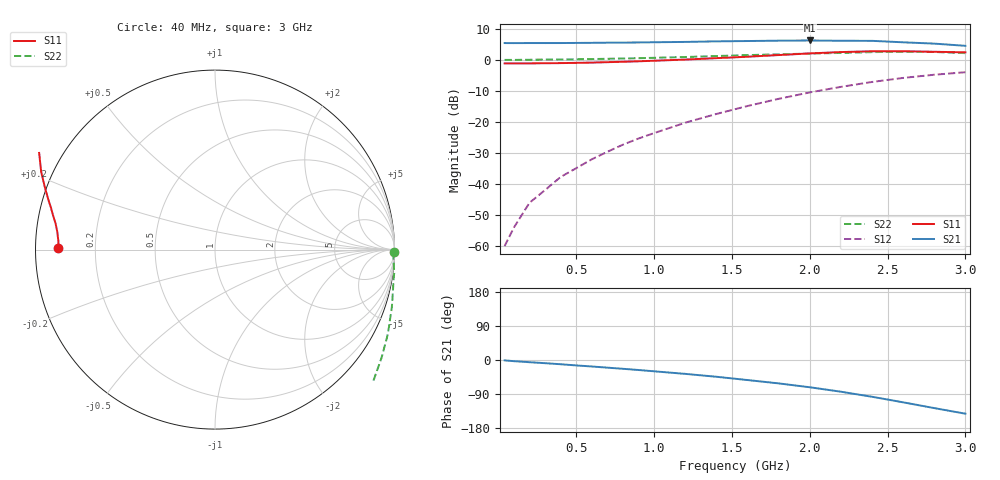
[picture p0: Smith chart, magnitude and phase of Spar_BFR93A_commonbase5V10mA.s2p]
! Filename:  BFR93ACB.S2P  Version:  2.0
! NXP part #: BFR93A  Date: Jul 1990
! Bias condition: Vce=5V, Ic=10mA
! COMMON BASE
#  MHz  S  MA  R  50
! Freq  S11  S21  S12  S22
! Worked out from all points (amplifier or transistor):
!   21 points, 40 MHz to 3 GHz, reference 50 ohm
!   highest |S21| = 6.2 dB at 2 GHz (marker M1)
!   |S21| within 3 dB of that: start of sweep to end of sweep
!   unconditionally stable (mu >= 1): nowhere
!   at 300 MHz: K = -0.60, MSG = 23.7 dB, |S12| = -41.9 dB
!   at 1 GHz: K = -0.92, MSG = 14.6 dB, |S12| = -23.6 dB
!   at 3 GHz: K = -0.70, MSG = 4.2 dB, |S12| = -4.0 dB
40  0.874 179.4  1.856 -1.0  0.001 67.4  0.995 -0.9
100  0.873 178.2  1.853 -3.1  0.002 85.9  0.995 -2.7
200  0.874 176.8  1.857 -5.8  0.005 106.2  1 -4.9
300  0.879 175.2  1.856 -8.4  0.008 120.1  1.007 -7.5
400  0.883 173.8  1.857 -11.2  0.013 129.3  1.01 -10.1
500  0.891 172.3  1.865 -14.3  0.018 135.0  1.017 -12.8
600  0.9 170.7  1.872 -17.1  0.025 137.5  1.026 -15.5
700  0.914 169.0  1.882 -20.2  0.033 140.2  1.037 -18.2
800  0.928 167.4  1.888 -23.2  0.043 141.2  1.047 -21.1
900  0.944 165.6  1.898 -26.4  0.054 142.2  1.06 -23.8
1000  0.964 163.8  1.912 -29.8  0.066 142.0  1.075 -26.8
1200  1.007 160.1  1.936 -36.6  0.097 141.6  1.107 -33.1
1400  1.061 155.9  1.977 -44.2  0.134 139.1  1.148 -39.9
1600  1.118 151.2  2.001 -52.9  0.18 136.4  1.188 -47.2
1800  1.19 145.7  2.027 -61.7  0.235 131.6  1.224 -55.6
2000  1.264 139.6  2.044 -71.9  0.298 126.1  1.257 -65.0
2200  1.33 133.3  2.019 -83.7  0.366 119.5  1.287 -76.2
2400  1.368 125.6  2.015 -97.0  0.439 111.5  1.326 -88.1
2600  1.369 117.2  1.909 -111.7  0.51 103.2  1.345 -99.8
2800  1.344 107.4  1.818 -126.9  0.574 94.1  1.333 -111.5
3000  1.316 97.9  1.676 -141.7  0.63 86.4  1.277 -122.8
